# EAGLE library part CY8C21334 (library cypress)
PSoC® Programmable System-on-Chip? M8C Processor Speeds to 24 MHz Source: http://www.cypress.com .. 38-12025_0P_V.pdf
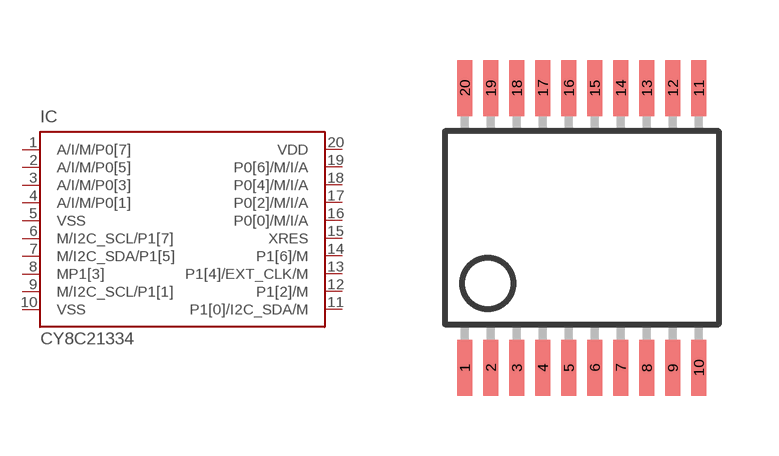
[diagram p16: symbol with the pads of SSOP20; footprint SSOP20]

Designator prefix IC

## CY8C21334 (MPN: CY8C21334-12PVXE; OC_FARNELL: 1321731; OC_NEWARK: 53M3699)  [SSOP20]
1  A/I/M/P0[7]
2  A/I/M/P0[5]
3  A/I/M/P0[3]
4  A/I/M/P0[1]
5  VSS  pwr
6  M/I2C_SCL/P1[7]
7  M/I2C_SDA/P1[5]
8  MP1[3]
9  M/I2C_SCL/P1[1]
10  VSS  pwr
11  P1[0]/I2C_SDA/M
12  P1[2]/M
13  P1[4]/EXT_CLK/M
14  P1[6]/M
15  XRES  in
16  P0[0]/M/I/A
17  P0[2]/M/I/A
18  P0[4]/M/I/A
19  P0[6]/M/I/A
20  VDD  pwr

## Footprint SSOP20 (pad centres in mm)
Small Shrink Outline Package 20-Pin (210-MIL) SSOP Source: http://www.cypress.com .. 38-12025_0P_V.pdf
smd 0.38 x 1.4: 1 -2.925,-3.5; 2 -2.275,-3.5; 3 -1.625,-3.5; 4 -0.975,-3.5; 5 -0.325,-3.5; 6 0.325,-3.5; 7 0.975,-3.5; 8 1.625,-3.5; 9 2.275,-3.5; 10 2.925,-3.5; 11 2.925,3.5; 12 2.275,3.5; 13 1.625,3.5; 14 0.975,3.5; 15 0.325,3.5; 16 -0.325,3.5; 17 -0.975,3.5; 18 -1.625,3.5; 19 -2.275,3.5; 20 -2.925,3.5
